
DATA_BLOCK DB3503
TITLE=
VERSION : 0.1

STRUCT
   CM_ID : STRING  [8 ] := '=PRM'; //COMPOSITE MACHINE
   STATION_ID : STRING  [8 ] := '++OP10'; //STATION - TRATTO - ZONE
   ELEMENT_ID : STRING  [8 ] := '+82CLM82'; //ELEMENT
   DB_ID : INT := 0 ; //DB SIZE OR TYPE
   PART_STYLE : STRING  [12 ]; //PART STYLE ON LAST STATION
   ACT_CYCLE_TIME : INT ; //ACTUAL CYCLE TIME FOR THIS STYLE
   COUNT_GOOD : INT ; //COUNTER GOOD PIECES
   COUNT_SCRAP : INT ; //COUNTER SCRAP PIECES
   SPARE_00 : ARRAY  [0 .. 15 ] OF //SPARE INTEGER
   INT ;
   SPARE_01 : ARRAY  [0 .. 17 ] OF //SPARE INTEGER
   INT ;
   CODE_EVENT : ARRAY  [0 .. 7 ] OF //CODE EVENT - EXTENDED FAULT CODE DIAGNOSTIC
   INT ;
   EVENT : STRUCT
E0000 : BOOL ; //+82CLM82-B49N_TEMP;MS.GENERALI ERRORE;1
E0001 : BOOL ; //+82CLM82-B49N_TEMP;MS.GENERALI AVVERTIMENTO;2
E0002 : BOOL ; //+82CLM82-B49N_TEMP; MS.  TEMPERATURA OK;58
E0003 : BOOL ; //+82CLM82-B49N_TEMP; MS. MS_03;58
E0004 : BOOL ; //+82CLM82-B49N_TEMP; MS. MS_04;58
E0005 : BOOL ; //+82CLM82-B49N_TEMP; MS. MS_05;58
E0006 : BOOL ; //+82CLM82-B49N_TEMP; MS. MS_06;58
E0007 : BOOL ; //+82CLM82-B49N_TEMP; MS. MS_07;58
E0008 : BOOL ; //+82CLM82-B49N_TEMP;MS.L03 MASSIMO AVVERTIMENTO;2
E0009 : BOOL ; //+82CLM82-B49N_TEMP;MS.L02 MINIMO AVVERTIMENTO;2
E0010 : BOOL ; //+82CLM82-B49N_TEMP; MS. MS_12;58
E0011 : BOOL ; //+82CLM82-B49N_TEMP; MS. MS_13;58
E0012 : BOOL ; //+82CLM82-B49N_TEMP; MS. MS_14;58
E0013 : BOOL ; //+82CLM82-B49N_TEMP; MS. MS_15;58
E0014 : BOOL ; //+82CLM82-B49N_TEMP; MS. MS_16;58
E0015 : BOOL ; //+82CLM82-B49N_TEMP; MS. TEMPERATURA TROPPO ALTA;58
E0016 : BOOL ; //+82CLM82-B49N_TEMP;ME.L04 MASSIMO ERRORE;1
E0017 : BOOL ; //+82CLM82-B49N_TEMP;ME.L01 MINIMO ERRORE;1
E0018 : BOOL ; //+82CLM82-B49N_TEMP; ME. ME_02;58
E0019 : BOOL ; //+82CLM82-B49N_TEMP; ME. ME_03;58
E0020 : BOOL ; //+82CLM82-B49N_TEMP; ME. ME_04;58
E0021 : BOOL ; //+82CLM82-B49N_TEMP; ME. ME_05;58
E0022 : BOOL ; //+82CLM82-B49N_TEMP; ME. ME_06;58
E0023 : BOOL ; //+82CLM82-B49N_TEMP; ME. ME_07;58
E0024 : BOOL ; //+82CLM82-B49N_TEMP; ME. ME_10;58
E0025 : BOOL ; //+82CLM82-B49N_TEMP; ME. ME_11;58
E0026 : BOOL ; //+82CLM82-B49N_TEMP; ME. ME_12;58
E0027 : BOOL ; //+82CLM82-B49N_TEMP; ME. ME_13;58
E0028 : BOOL ; //+82CLM82-B49N_TEMP; ME. ME_14;58
E0029 : BOOL ; //+82CLM82-B49N_TEMP; ME. ME_15;58
E0030 : BOOL ; //+82CLM82-B49N_TEMP; ME. ME_16;58
E0031 : BOOL ; //+82CLM82-B49N_TEMP; ME. ME_17;58
E0032 : BOOL ; //+82CLM82-B49N_HUM;MS.GENERALI ERRORE;1
E0033 : BOOL ; //+82CLM82-B49N_HUM;MS.GENERALI AVVERTIMENTO;2
E0034 : BOOL ; //+82CLM82-B49N_HUM; MS.  TEMPERATURA OK;58
E0035 : BOOL ; //+82CLM82-B49N_HUM; MS. MS_03;58
E0036 : BOOL ; //+82CLM82-B49N_HUM; MS. MS_04;58
E0037 : BOOL ; //+82CLM82-B49N_HUM; MS. MS_05;58
E0038 : BOOL ; //+82CLM82-B49N_HUM; MS. MS_06;58
E0039 : BOOL ; //+82CLM82-B49N_HUM; MS. MS_07;58
E0040 : BOOL ; //+82CLM82-B49N_HUM;MS.L03 MASSIMO AVVERTIMENTO;2
E0041 : BOOL ; //+82CLM82-B49N_HUM;MS.L02 MINIMO AVVERTIMENTO;2
E0042 : BOOL ; //+82CLM82-B49N_HUM; MS. MS_12;58
E0043 : BOOL ; //+82CLM82-B49N_HUM; MS. MS_13;58
E0044 : BOOL ; //+82CLM82-B49N_HUM; MS. MS_14;58
E0045 : BOOL ; //+82CLM82-B49N_HUM; MS. MS_15;58
E0046 : BOOL ; //+82CLM82-B49N_HUM; MS. MS_16;58
E0047 : BOOL ; //+82CLM82-B49N_HUM; MS. TEMPERATURA TROPPO ALTA;58
E0048 : BOOL ; //+82CLM82-B49N_HUM;ME.L04 MASSIMO ERRORE;1
E0049 : BOOL ; //+82CLM82-B49N_HUM;ME.L01 MINIMO ERRORE;1
E0050 : BOOL ; //+82CLM82-B49N_HUM; ME. ME_02;58
E0051 : BOOL ; //+82CLM82-B49N_HUM; ME. ME_03;58
E0052 : BOOL ; //+82CLM82-B49N_HUM; ME. ME_04;58
E0053 : BOOL ; //+82CLM82-B49N_HUM; ME. ME_05;58
E0054 : BOOL ; //+82CLM82-B49N_HUM; ME. ME_06;58
E0055 : BOOL ; //+82CLM82-B49N_HUM; ME. ME_07;58
E0056 : BOOL ; //+82CLM82-B49N_HUM; ME. ME_10;58
E0057 : BOOL ; //+82CLM82-B49N_HUM; ME. ME_11;58
E0058 : BOOL ; //+82CLM82-B49N_HUM; ME. ME_12;58
E0059 : BOOL ; //+82CLM82-B49N_HUM; ME. ME_13;58
E0060 : BOOL ; //+82CLM82-B49N_HUM; ME. ME_14;58
E0061 : BOOL ; //+82CLM82-B49N_HUM; ME. ME_15;58
E0062 : BOOL ; //+82CLM82-B49N_HUM; ME. ME_16;58
E0063 : BOOL ; //+82CLM82-B49N_HUM; ME. ME_17;58
END_STRUCT;
END_STRUCT;
BEGIN
CM_ID := '=PRM';
STATION_ID := '++OP10';
ELEMENT_ID := '+82CLM82';
DB_ID := 0 ;
PART_STYLE := '';
ACT_CYCLE_TIME := 0;
COUNT_GOOD := 0;
COUNT_SCRAP := 0;
SPARE_00[0] := 0;
SPARE_00[1] := 0;
SPARE_00[2] := 0;
SPARE_00[3] := 0;
SPARE_00[4] := 0;
SPARE_00[5] := 0;
SPARE_00[6] := 0;
SPARE_00[7] := 0;
SPARE_00[8] := 0;
SPARE_00[9] := 0;
SPARE_00[10] := 0;
SPARE_00[11] := 0;
SPARE_00[12] := 0;
SPARE_00[13] := 0;
SPARE_00[14] := 0;
SPARE_00[15] := 0;
SPARE_01[0] := 0;
SPARE_01[1] := 0;
SPARE_01[2] := 0;
SPARE_01[3] := 0;
SPARE_01[4] := 0;
SPARE_01[5] := 0;
SPARE_01[6] := 0;
SPARE_01[7] := 0;
SPARE_01[8] := 0;
SPARE_01[9] := 0;
SPARE_01[10] := 0;
SPARE_01[11] := 0;
SPARE_01[12] := 0;
SPARE_01[13] := 0;
SPARE_01[14] := 0;
SPARE_01[15] := 0;
SPARE_01[16] := 0;
SPARE_01[17] := 0;
CODE_EVENT[0] := 0;
CODE_EVENT[1] := 0;
CODE_EVENT[2] := 0;
CODE_EVENT[3] := 0;
CODE_EVENT[4] := 0;
CODE_EVENT[5] := 0;
CODE_EVENT[6] := 0;
CODE_EVENT[7] := 0;
EVENT.E0000 := FALSE;
EVENT.E0001 := FALSE;
EVENT.E0002 := FALSE;
EVENT.E0003 := FALSE;
EVENT.E0004 := FALSE;
EVENT.E0005 := FALSE;
EVENT.E0006 := FALSE;
EVENT.E0007 := FALSE;
EVENT.E0008 := FALSE;
EVENT.E0009 := FALSE;
EVENT.E0010 := FALSE;
EVENT.E0011 := FALSE;
EVENT.E0012 := FALSE;
EVENT.E0013 := FALSE;
EVENT.E0014 := FALSE;
EVENT.E0015 := FALSE;
EVENT.E0016 := FALSE;
EVENT.E0017 := FALSE;
EVENT.E0018 := FALSE;
EVENT.E0019 := FALSE;
EVENT.E0020 := FALSE;
EVENT.E0021 := FALSE;
EVENT.E0022 := FALSE;
EVENT.E0023 := FALSE;
EVENT.E0024 := FALSE;
EVENT.E0025 := FALSE;
EVENT.E0026 := FALSE;
EVENT.E0027 := FALSE;
EVENT.E0028 := FALSE;
EVENT.E0029 := FALSE;
EVENT.E0030 := FALSE;
EVENT.E0031 := FALSE;
EVENT.E0032 := FALSE;
EVENT.E0033 := FALSE;
EVENT.E0034 := FALSE;
EVENT.E0035 := FALSE;
EVENT.E0036 := FALSE;
EVENT.E0037 := FALSE;
EVENT.E0038 := FALSE;
EVENT.E0039 := FALSE;
EVENT.E0040 := FALSE;
EVENT.E0041 := FALSE;
EVENT.E0042 := FALSE;
EVENT.E0043 := FALSE;
EVENT.E0044 := FALSE;
EVENT.E0045 := FALSE;
EVENT.E0046 := FALSE;
EVENT.E0047 := FALSE;
EVENT.E0048 := FALSE;
EVENT.E0049 := FALSE;
EVENT.E0050 := FALSE;
EVENT.E0051 := FALSE;
EVENT.E0052 := FALSE;
EVENT.E0053 := FALSE;
EVENT.E0054 := FALSE;
EVENT.E0055 := FALSE;
EVENT.E0056 := FALSE;
EVENT.E0057 := FALSE;
EVENT.E0058 := FALSE;
EVENT.E0059 := FALSE;
EVENT.E0060 := FALSE;
EVENT.E0061 := FALSE;
EVENT.E0062 := FALSE;
EVENT.E0063 := FALSE;
END_DATA_BLOCK
